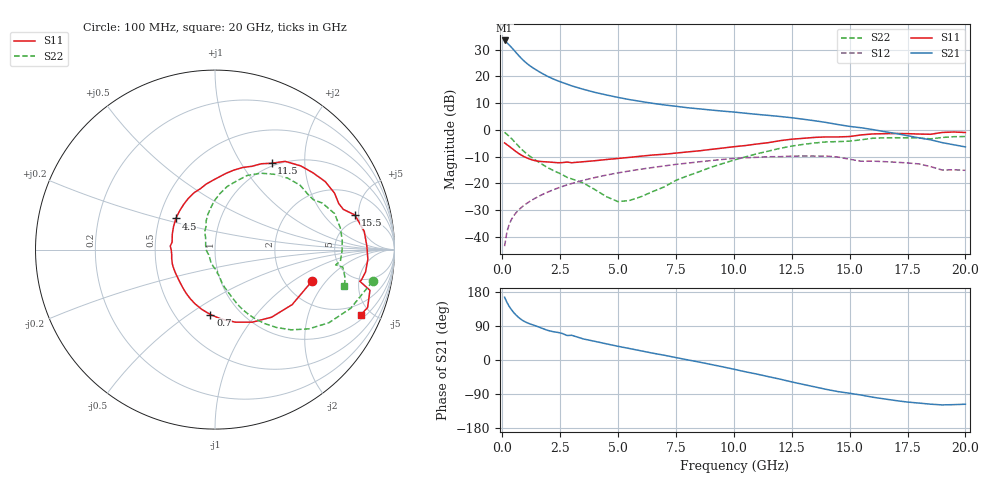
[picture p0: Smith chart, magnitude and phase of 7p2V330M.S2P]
! Infineon Technologies  Discrete & RF Semiconductors
! bfp620
! VCE =  2.3 V,  IC =  30 mA
! Common Emitter S-Parameters:  Sep 2002
# GHz  S  MA  R  50
!  f  S11  S21  S12  S22
! GHz  MAG  ANG  MAG  ANG  MAG  ANG  MAG  ANG
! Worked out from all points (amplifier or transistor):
!   59 points, 100 MHz to 20 GHz, reference 50 ohm
!   highest |S21| = 33.4 dB at 100 MHz (marker M1)
!   |S21| within 3 dB of that: start of sweep to 439.4 MHz
!   unconditionally stable (mu >= 1): 2.868 GHz to 9.906 GHz; 17.18 GHz to end of sweep
!   at 1 GHz: K = 0.79, MSG = 26.6 dB, |S12| = -27.9 dB
!   at 5.5 GHz: K = 1.04, MAG = 12.1 dB, |S12| = -15.4 dB
!   at 20 GHz: K = 1.25, MAG = 1.3 dB, |S12| = -15.1 dB
!   S11 on the Smith chart (normalised r, x): 100 MHz: 2.82, -1.45; 700 MHz: 0.73, -0.61; 4.5 GHz: 0.61, +0.23; 11.5 GHz: 0.96, +1.38; 15.5 GHz: 4.14, +4.49; 20 GHz: 1.25, -4.36
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0.1  0.5695 -17.7  46.68 165.7  0.0067 61.3  0.8955 -11.4
0.2  0.5279 -35.5  42.33 152.1  0.0124 64.5  0.8238 -23.4
0.3  0.4912 -50.1  38.38 141.3  0.0172 64.1  0.7543 -32.7
0.4  0.4548 -62.7  34.54 132.4  0.0213 63.1  0.6842 -40.2
0.5  0.4202 -74.2  30.88 124.8  0.025 62.1  0.6161 -46.5
0.6  0.3893 -84.6  27.55 118.2  0.0284 61.3  0.553 -51.7
0.7  0.3628 -94.1  24.62 112.6  0.0316 60.6  0.4967 -56.1
0.8  0.3407 -102.6  22.13 107.7  0.0347 60.1  0.4482 -59.7
1  0.3065 -116.7  18.3 100.3  0.0405 59.5  0.3726 -64.9
1.2  0.2823 -127.9  15.64 95.2  0.0463 59.0  0.319 -68.2
1.6  0.2575 -146.4  12.12 86.5  0.0579 57.6  0.2448 -73.1
2.2  0.2462 -168.4  8.911 74.7  0.0756 54.3  0.1738 -79.2
2.8  0.25 175.5  7.117 64.6  0.0935 50.1  0.1293 -85.0
3.5  0.2533 159.9  5.712 55.6  0.1141 44.4  0.1015 -92.5
4.5  0.2786 141.5  4.473 42.6  0.1428 35.8  0.0563 -120.7
7  0.3494 103.3  2.914 12.5  0.2116 12.7  0.086 127.5
10.5  0.5082 66.0  2.04 -31.1  0.3001 -26.1  0.3116 85.2
11.5  0.5757 56.7  1.858 -44.0  0.314 -38.1  0.4004 72.6
13.5  0.7216 31.7  1.475 -71.0  0.3231 -62.1  0.5677 44.6
15.5  0.8028 13.9  1.091 -92.5  0.2589 -84.1  0.6514 23.5
17  0.8534 -3.6  0.853 -107.1  0.2477 -94.1  0.711 4.3
20  0.8902 -24.0  0.479 -116.7  0.1749 -103.8  0.7477 -15.7
